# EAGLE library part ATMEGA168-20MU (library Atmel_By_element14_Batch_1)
8-bit Microcontroller with In-System Programmable Flash
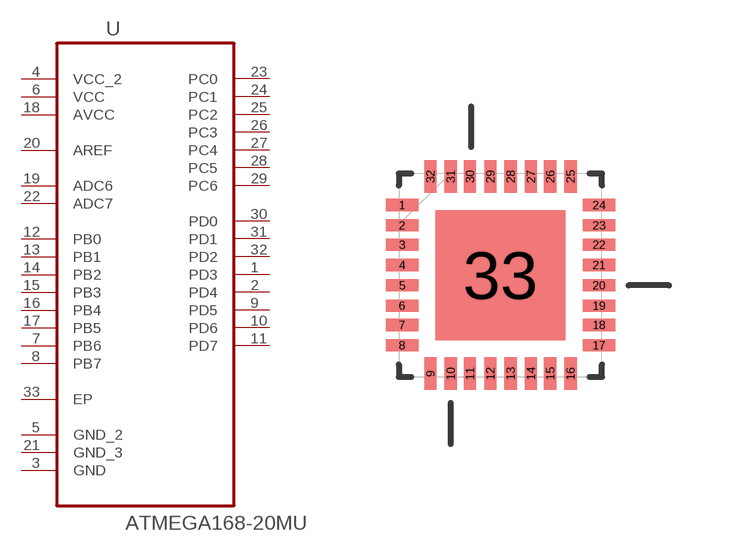
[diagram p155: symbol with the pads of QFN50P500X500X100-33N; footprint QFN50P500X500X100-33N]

Designator prefix U

## ATMEGA168-20MU (MPN: ATMEGA168-20MU; OC_FARNELL: 1455105; OC_NEWARK: 58M3731; PACKAGE: QFN-32; SUPPLIER: Atmel)  [QFN50P500X500X100-33N]
1  PD3
2  PD4
3  GND  pas
4  VCC_2  pwr
5  GND_2  pas
6  VCC  pwr
7  PB6
8  PB7
9  PD5
10  PD6
11  PD7
12  PB0
13  PB1
14  PB2
15  PB3
16  PB4
17  PB5
18  AVCC  pwr
19  ADC6  in
20  AREF  in
21  GND_3  pas
22  ADC7  in
23  PC0
24  PC1
25  PC2
26  PC3
27  PC4
28  PC5
29  PC6
30  PD0
31  PD1
32  PD2
33  EP  pas

## Footprint QFN50P500X500X100-33N (pad centres in mm)
smd 0.813 x 0.305: 1 -2.464,1.753; 2 -2.464,1.245; 3 -2.464,0.762; 4 -2.464,0.254; 5 -2.464,-0.254; 6 -2.464,-0.762; 7 -2.464,-1.245; 8 -2.464,-1.753; 17 2.464,-1.753; 18 2.464,-1.245; 19 2.464,-0.762; 20 2.464,-0.254; 21 2.464,0.254; 22 2.464,0.762; 23 2.464,1.245; 24 2.464,1.753
smd 0.305 x 0.813: 9 -1.753,-2.464; 10 -1.245,-2.464; 11 -0.762,-2.464; 12 -0.254,-2.464; 13 0.254,-2.464; 14 0.762,-2.464; 15 1.245,-2.464; 16 1.753,-2.464; 25 1.753,2.464; 26 1.245,2.464; 27 0.762,2.464; 28 0.254,2.464; 29 -0.254,2.464; 30 -0.762,2.464; 31 -1.245,2.464; 32 -1.753,2.464
smd 3.251 x 3.251: 33 0,0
